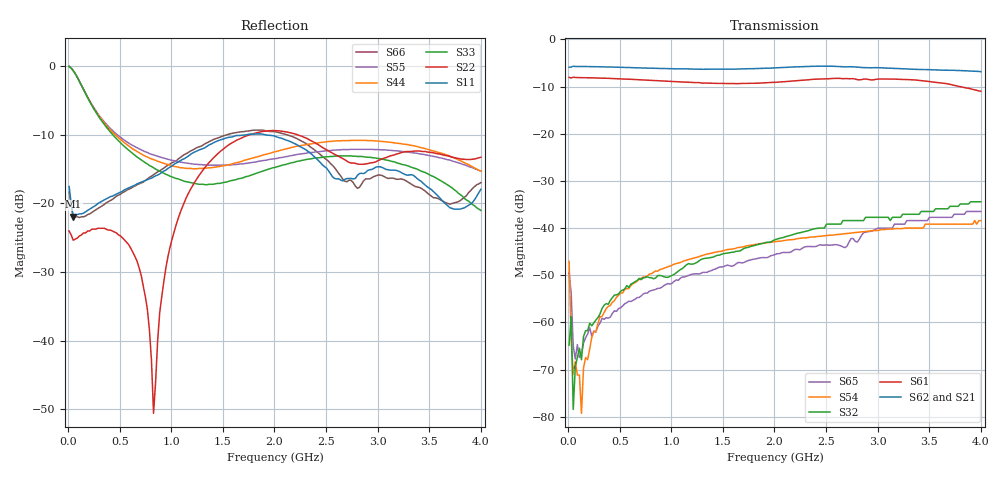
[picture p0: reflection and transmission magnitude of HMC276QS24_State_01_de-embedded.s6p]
! Hittite Microwave Corporation
! 20 Alpha Road
! Chelmsford, MA 01824
! Tel: 978-250-3343
! Fax: 978-250-3373
! Device: HMC276QS24, 0.7-3.0 GHz, GaAS MMIC 4x2 Switch Matrix in 24-lead QSOP package
! Misc: Data was de-embedded to package pins.
!  Port 1 = OP1
!  Port 2 = VL
!  Port 3 = VH
!  Port 4 = HH
!  Port 5 = HL
!  Port 6 = OP2
!  Vdd = +5 V
!  Vctl = 0 V[Logic 0] / +5 V[Logic 1]
!  State 01,  VL to OP1,  VL to OP2
!  Control Lines (Logic)
!  HV 1 = 0, Tone 1 = 0
!  HV 2 = 0, Tone 2 = 0
!  Data reformated to new Touchstone file format - Wed Jan 10 10:45:23 2007
# MHz S DB R 50
! 6 Port Network Data
! freq  dbS11  angS11  dbS12  angS12  dbS13  angS13  dbS14  angS14
!  dbS15  angS15  dbS16  angS16
!  dbS21  angS21  dbS22  angS22
!  dbS23  angS23  dbS24  angS24  dbS25  angS25  dbS26  angS26
!  dbS31  angS31  dbS32  angS32  dbS33  angS33  dbS34  angS34
!  dbS35  angS35  dbS36  angS36
!  dbS41  angS41  dbS42  angS42
!  dbS43  angS43  dbS44  angS44  dbS45  angS45  dbS46  angS46
!  dbS51  angS51  dbS52  angS52  dbS53  angS53  dbS54  angS54
!  dbS55  angS55  dbS56  angS56
!  dbS61  angS61  dbS62  angS62
!  dbS63  angS63  dbS64  angS64  dbS65  angS65  dbS66  angS66
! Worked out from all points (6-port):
!   201 points, 10 MHz to 4 GHz, reference 50 ohm
!   strongest paths, dB at 10 MHz, 1.008 GHz, 2.005 GHz, 3.002 GHz, 4 GHz:
!     S62: -5.9, -6.2, -6.0, -6.0, -6.8
!     S21: -5.7, -6.2, -6.0, -6.1, -6.9
!     S61: -8.0, -8.9, -9.1, -8.4, -11.0
!     S32: -64.8, -50.1, -42.5, -37.7, -34.4
!     S54: -47.1, -47.9, -42.9, -40.5, -38.4
!     S65: -49.6, -51.7, -45.6, -40.0, -36.5
!   lowest |S11| = -21.9 dB at 49.9 MHz (marker M1), VSWR 1.17, Z = 58 - j3.2 ohm
!   |S11| at or under -10 dB: start of sweep to 1.727 GHz; 1.913 GHz to end of sweep
